| IBIS file stm32u3b5_3c5_ufqfpn48.ibs
| Created by kronos
| SIEMENS-EDA 2024.1_2
[IBIS ver] 4.2
[File name] stm32u3b5_3c5_ufqfpn48.ibs
[File Rev] 0.1
[Date] 09-03-2026
[Source] Data Created at STMicroelectronics
[Notes]  File originated from ELDO simulations.
[Disclaimer]  This information is for modeling purpose only and is
   not guaranted. The information is subject to change without
   notice.
[Copyright] Copyright 2026 STMicroelectronics Inc.
|   Component stm32u3b5_3c5_ufqfpn48
[Component] stm32u3b5_3c5_ufqfpn48
[Manufacturer] STMicroelectronics
[Package]
| variable   typ   min   max
R_pkg  0  NA  NA
L_pkg  0  NA  NA
C_pkg  0  NA  NA
[Pin]   signal_name   model_name
0  VSS  gnd
1  VBAT  power
2  PC13  io8_ft_100m_v33
3  PC14-OSC32_IN  io_ft_tamp
4  PC15-OSC32_OUT  io_ft_tamp
5  PH0-OSC_IN  io8_ft_100m
6  PH1-OSC_OUT  io8_ft_100m
7  NRST  ioreset_v33
8  VSSA  nc
9  VDDA  nc
10  PA0  io8_ft_100m
11  PA1  io8_ft_100m_hslv
12  PA2  io8_ft_100m_hslv
13  PA3  io8_ft_100m_hslv
14  PA4  io8_ft_100m_hslv
15  PA5  io8_ft_100m
16  PA6  io8_ft_100m_hslv
17  PA7  io8_ft_100m_hslv
18  PB0  io8_ft_100m_hslv
19  PB1  io8_ft_100m_hslv
20  PB2  io8_ft_100m_hslv
21  PB10  io8_ft_100m_hslv
22  VDD11  nc
23  VSS  gnd
24  VDD  power
25  PB12  io8_ft_100m_hslv
26  PB13  io8_ft_100m_hslv
27  PB14  io8_ft_100m_hslv
28  PB15  io8_ft_100m
29  PA8  io8_ft_100m_hslv
30  PA9  io8_ft_100m
31  PA10  io8_ft_100m
32  PA11  io8usb_ft_phy
33  PA12  io8usb_ft_phy
34  PA13  io8_ft_100m
35  VSS  gnd
36  VDD  power
37  PA14  io8_ft_100m
38  PA15  io8_ft_100m
39  PB3  io8_ft_100m_hslv
40  PB4  io8_ft_100m_hslv
41  PB5  io8_ft_100m_hslv
42  PB6  io8_ft_100m_hslv
43  PB7  io8_ft_100m_hslv
44  PH3-BOOT0  io8_ft_100m_hslv
45  PB8  io8_ft_100m_hslv
46  PB9  io8_ft_100m_hslv
47  VSS  gnd
48  VDD  power
[Package Model]   42a-ufqfpn-7x7-48-260217
[Pin Mapping]   pulldown_ref   pullup_ref   | Comment
0  gndio  nc
1  nc  vsw
2  gndio  vsw
3  gndio  vsw
4  gndio  vsw
5  gndio  vddio
6  gndio  vddio
7  gndio  vddio
8  nc  nc
9  nc  nc
10  gndio  vddio
11  gndio  vddio
12  gndio  vddio
13  gndio  vddio
14  gndio  vddio
15  gndio  vddio
16  gndio  vddio
17  gndio  vddio
18  gndio  vddio
19  gndio  vddio
20  gndio  vddio
21  gndio  vddio
22  nc  nc
23  gndio  nc
24  nc  vddio
25  gndio  vddio
26  gndio  vddio
27  gndio  vddio
28  gndio  vddio
29  gndio  vddio
30  gndio  vddio
31  gndio  vddio
32  gndio  vddio
33  gndio  vddio
34  gndio  vddio
35  gndio  nc
36  nc  vddio
37  gndio  vddio
38  gndio  vddio
39  gndio  vddio
40  gndio  vddio
41  gndio  vddio
42  gndio  vddio
43  gndio  vddio
44  gndio  vddio
45  gndio  vddio
46  gndio  vddio
47  gndio  nc
48  nc  vddio
|[Diff Pin]  inv_pin  vdiff  tdelay_typ  tdelay_min  tdelay_max
|33  32  NA  NA  NA  NA
[Model Selector] io8_ft_100m
io8_ft_100m_ls_1v2  "GPIO 100MHz - 5V tolerant - low speed - 1.2V range"
io8_ft_100m_ls_1v8  "GPIO 100MHz - 5V tolerant - low speed - 1.8V range"
io8_ft_100m_ls_3v3  "GPIO 100MHz - 5V tolerant - low speed - 3.3V range"
io8_ft_100m_ms_1v2  "GPIO 100MHz - 5V tolerant - med speed - 1.2V range"
io8_ft_100m_ms_1v8  "GPIO 100MHz - 5V tolerant - med speed - 1.8V range"
io8_ft_100m_ms_3v3  "GPIO 100MHz - 5V tolerant - med speed - 3.3V range"
io8_ft_100m_fs_1v2  "GPIO 100MHz - 5V tolerant - fast speed - 1.2V range"
io8_ft_100m_fs_1v8  "GPIO 100MHz - 5V tolerant - fast speed - 1.8V range"
io8_ft_100m_fs_3v3  "GPIO 100MHz - 5V tolerant - fast speed - 3.3V range"
io8_ft_100m_hs_1v2  "GPIO 100MHz - 5V tolerant - high speed - 1.2V range"
io8_ft_100m_hs_1v8  "GPIO 100MHz - 5V tolerant - high speed - 1.8V range"
io8_ft_100m_hs_3v3  "GPIO 100MHz - 5V tolerant - high speed - 3.3V range"
[Model Selector] io8_ft_100m_hslv
io8_ft_100m_ls_1v2  "GPIO 100MHz - 5V tolerant - low speed - 1.2V range"
io8_ft_100m_ls_1v8  "GPIO 100MHz - 5V tolerant - low speed - 1.8V range"
io8_ft_100m_ls_3v3  "GPIO 100MHz - 5V tolerant - low speed - 3.3V range"
io8_ft_100m_ms_1v2  "GPIO 100MHz - 5V tolerant - med speed - 1.2V range"
io8_ft_100m_ms_1v8  "GPIO 100MHz - 5V tolerant - med speed - 1.8V range"
io8_ft_100m_ms_3v3  "GPIO 100MHz - 5V tolerant - med speed - 3.3V range"
io8_ft_100m_fs_1v2  "GPIO 100MHz - 5V tolerant - fast speed - 1.2V range"
io8_ft_100m_fs_1v8  "GPIO 100MHz - 5V tolerant - fast speed - 1.8V range"
io8_ft_100m_fs_3v3  "GPIO 100MHz - 5V tolerant - fast speed - 3.3V range"
io8_ft_100m_hs_1v2  "GPIO 100MHz - 5V tolerant - high speed - 1.2V range"
io8_ft_100m_hs_1v8  "GPIO 100MHz - 5V tolerant - high speed - 1.8V range"
io8_ft_100m_hs_3v3  "GPIO 100MHz - 5V tolerant - high speed - 3.3V range"
io8_ft_100m_hslv_ls_1v2  "GPIO 100MHz low voltage optimization - 5V tolerant - low speed - 1.2V range"
io8_ft_100m_hslv_ls_1v8  "GPIO 100MHz low voltage optimization - 5V tolerant - low speed - 1.8V range"
io8_ft_100m_hslv_ls_2v5  "GPIO 100MHz low voltage optimization - 5V tolerant - low speed - 3.3V range"
io8_ft_100m_hslv_ms_1v2  "GPIO 100MHz low voltage optimization - 5V tolerant - med speed - 1.2V range"
io8_ft_100m_hslv_ms_1v8  "GPIO 100MHz low voltage optimization - 5V tolerant - med speed - 1.8V range"
io8_ft_100m_hslv_ms_2v5  "GPIO 100MHz low voltage optimization - 5V tolerant - med speed - 3.3V range"
io8_ft_100m_hslv_fs_1v2  "GPIO 100MHz low voltage optimization - 5V tolerant - fast speed - 1.2V range"
io8_ft_100m_hslv_fs_1v8  "GPIO 100MHz low voltage optimization - 5V tolerant - fast speed - 1.8V range"
io8_ft_100m_hslv_fs_2v5  "GPIO 100MHz low voltage optimization - 5V tolerant - fast speed - 3.3V range"
io8_ft_100m_hslv_hs_1v2  "GPIO 100MHz low voltage optimization - 5V tolerant - high speed - 1.2V range"
io8_ft_100m_hslv_hs_1v8  "GPIO 100MHz low voltage optimization - 5V tolerant - high speed - 1.8V range"
io8_ft_100m_hslv_hs_2v5  "GPIO 100MHz low voltage optimization - 5V tolerant - high speed - 3.3V range"
[Model Selector] io8_ft_100m_v33
io8_ft_100m_v33_ls_1v2  "GPIO_V33 100MHz - 5V tolerant - low speed - 1.2V range"
io8_ft_100m_v33_ls_1v8  "GPIO_V33 100MHz - 5V tolerant - low speed - 1.8V range"
io8_ft_100m_v33_ls_3v3  "GPIO_V33 100MHz - 5V tolerant - low speed - 3.3V range"
io8_ft_100m_v33_ms_1v2  "GPIO_V33 100MHz - 5V tolerant - med speed - 1.2V range"
io8_ft_100m_v33_ms_1v8  "GPIO_V33 100MHz - 5V tolerant - med speed - 1.8V range"
io8_ft_100m_v33_ms_3v3  "GPIO_V33 100MHz - 5V tolerant - med speed - 3.3V range"
io8_ft_100m_v33_fs_1v2  "GPIO_V33 100MHz - 5V tolerant - fast speed - 1.2V range"
io8_ft_100m_v33_fs_1v8  "GPIO_V33 100MHz - 5V tolerant - fast speed - 1.8V range"
io8_ft_100m_v33_fs_3v3  "GPIO_V33 100MHz - 5V tolerant - fast speed - 3.3V range"
io8_ft_100m_v33_hs_1v2  "GPIO_V33 100MHz - 5V tolerant - high speed - 1.2V range"
io8_ft_100m_v33_hs_1v8  "GPIO_V33 100MHz - 5V tolerant - high speed - 1.8V range"
io8_ft_100m_v33_hs_3v3  "GPIO_V33 100MHz - 5V tolerant - high speed - 3.3V range"
[Model Selector] io8usb_ft_phy
io8_ft_100m_ls_1v2  "GPIO 100MHz - 5V tolerant - low speed - 1.2V range"
io8_ft_100m_ls_1v8  "GPIO 100MHz - 5V tolerant - low speed - 1.8V range"
io8_ft_100m_ls_3v3  "GPIO 100MHz - 5V tolerant - low speed - 3.3V range"
io8_ft_100m_ms_1v2  "GPIO 100MHz - 5V tolerant - med speed - 1.2V range"
io8_ft_100m_ms_1v8  "GPIO 100MHz - 5V tolerant - med speed - 1.8V range"
io8_ft_100m_ms_3v3  "GPIO 100MHz - 5V tolerant - med speed - 3.3V range"
io8_ft_100m_fs_1v2  "GPIO 100MHz - 5V tolerant - fast speed - 1.2V range"
io8_ft_100m_fs_1v8  "GPIO 100MHz - 5V tolerant - fast speed - 1.8V range"
io8_ft_100m_fs_3v3  "GPIO 100MHz - 5V tolerant - fast speed - 3.3V range"
io8_ft_100m_hs_1v2  "GPIO 100MHz - 5V tolerant - high speed - 1.2V range"
io8_ft_100m_hs_1v8  "GPIO 100MHz - 5V tolerant - high speed - 1.8V range"
io8_ft_100m_hs_3v3  "GPIO 100MHz - 5V tolerant - high speed - 3.3V range"
io8usb_ft_phy_hs_3v3   "USB full speed"
io8usb_ft_phy_ls_3v3   "USB low speed"
[Model Selector] io_ft_tamp
io_ft_tamp_ls_1v2 "io8_ft tamp low speed @ 1.2V"
io_ft_tamp_ls_1v8 "io8_ft tamp low speed @ 1.8V"
io_ft_tamp_ls_3v3 "io8_ft tamp low speed @ 3.3V"
io_ft_tamp_ms_1v2 "io8_ft tamp med speed @ 1.2V"
io_ft_tamp_ms_1v8 "io8_ft tamp med speed @ 1.8V"
io_ft_tamp_ms_3v3 "io8_ft tamp med speed @ 3.3V"
io_ft_tamp_fs_1v2 "io8_ft tamp fast speed @ 1.2V"
io_ft_tamp_fs_1v8 "io8_ft tamp fast speed @ 1.8V"
io_ft_tamp_fs_3v3 "io8_ft tamp fast speed @ 3.3V"
io_ft_tamp_hs_1v2 "io8_ft tamp high speed @ 1.2V"
io_ft_tamp_hs_1v8 "io8_ft tamp high speed @ 1.8V"
io_ft_tamp_hs_3v3 "io8_ft tamp high speed @ 3.3V"
[Model Selector] ioreset_v33
ioreset_v33_1v2 "Reset PAD. 5V tolerant. 1.2V range"
ioreset_v33_1v8 "Reset PAD. 5V tolerant. 1.8V range"
ioreset_v33_3v3 "Reset PAD. 5V tolerant. 3.3V range"
[Define Package Model]  42a-ufqfpn-7x7-48-260217
[Manufacturer]  Unknown
[OEM]  Unknown
[Description]  None
[Number Of Pins]  47
[Pin Numbers]
| Pin Num   Terminal Name
7 | NRST
10 | PA0
31 | PA10
32 | PA11
33 | PA12
34 | PA13
37 | PA14
38 | PA15
11 | PA1
12 | PA2
13 | PA3
14 | PA4
15 | PA5
16 | PA6
17 | PA7
29 | PA8
30 | PA9
18 | PB0
21 | PB10
25 | PB12
26 | PB13
27 | PB14
28 | PB15
19 | PB1
20 | PB2
39 | PB3
40 | PB4
41 | PB5
42 | PB6
43 | PB7
45 | PB8
46 | PB9
2 | PC13
3 | PC14-OSC32_IN
4 | PC15-OSC32_OUT
5 | PH0-OSC_IN
6 | PH1-OSC_OUT
44 | PH3-BOOT0
22 | VDD11
36 | VDD
48 | VDD
1 | VBAT
24 | VDD
9 | VDDA
0 | VSS
35 | VSS
8 | VSSA
|[Merged Pins]  0
|23  |  VSS
|47  |  VSS
[Model Data]
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[End Model Data]
[End Package Model]
|End [Component]
| Models and submodels in the file (53): io8_ft_100m_fs_1v2 (I/O), io8_ft_100m_fs_1v8 (I/O), io8_ft_100m_fs_3v3 (I/O), io8_ft_100m_hs_1v2 (I/O), io8_ft_100m_hs_1v8 (I/O), io8_ft_100m_hs_3v3 (I/O), io8_ft_100m_hslv_fs_1v2 (I/O), io8_ft_100m_hslv_fs_1v8 (I/O), io8_ft_100m_hslv_fs_2v5 (I/O), io8_ft_100m_hslv_hs_1v2 (I/O), io8_ft_100m_hslv_hs_1v8 (I/O), io8_ft_100m_hslv_hs_2v5 (I/O), io8_ft_100m_hslv_ls_1v2 (I/O), io8_ft_100m_hslv_ls_1v8 (I/O), io8_ft_100m_hslv_ls_2v5 (I/O), io8_ft_100m_hslv_ms_1v2 (I/O), io8_ft_100m_hslv_ms_1v8 (I/O), io8_ft_100m_hslv_ms_2v5 (I/O), io8_ft_100m_ls_1v2 (I/O), io8_ft_100m_ls_1v8 (I/O), io8_ft_100m_ls_3v3 (I/O), io8_ft_100m_ms_1v2 (I/O), io8_ft_100m_ms_1v8 (I/O), io8_ft_100m_ms_3v3 (I/O), io8_ft_100m_v33_fs_1v2 (I/O), io8_ft_100m_v33_fs_1v8 (I/O), io8_ft_100m_v33_fs_3v3 (I/O), io8_ft_100m_v33_hs_1v2 (I/O), io8_ft_100m_v33_hs_1v8 (I/O), io8_ft_100m_v33_hs_3v3 (I/O), io8_ft_100m_v33_ls_1v2 (I/O), io8_ft_100m_v33_ls_1v8 (I/O), io8_ft_100m_v33_ls_3v3 (I/O), io8_ft_100m_v33_ms_1v2 (I/O), io8_ft_100m_v33_ms_1v8 (I/O), io8_ft_100m_v33_ms_3v3 (I/O), io8usb_ft_phy_hs_3v3 (I/O), io8usb_ft_phy_ls_3v3 (I/O), io_ft_tamp_fs_1v2 (I/O), io_ft_tamp_fs_1v8 (I/O), io_ft_tamp_fs_3v3 (I/O), io_ft_tamp_hs_1v2 (I/O), io_ft_tamp_hs_1v8 (I/O), io_ft_tamp_hs_3v3 (I/O), io_ft_tamp_ls_1v2 (I/O), io_ft_tamp_ls_1v8 (I/O), io_ft_tamp_ls_3v3 (I/O), io_ft_tamp_ms_1v2 (I/O), io_ft_tamp_ms_1v8 (I/O), io_ft_tamp_ms_3v3 (I/O), ioreset_v33_1v2 (I/O_open_drain), ioreset_v33_1v8 (I/O_open_drain), ioreset_v33_3v3 (I/O_open_drain)
